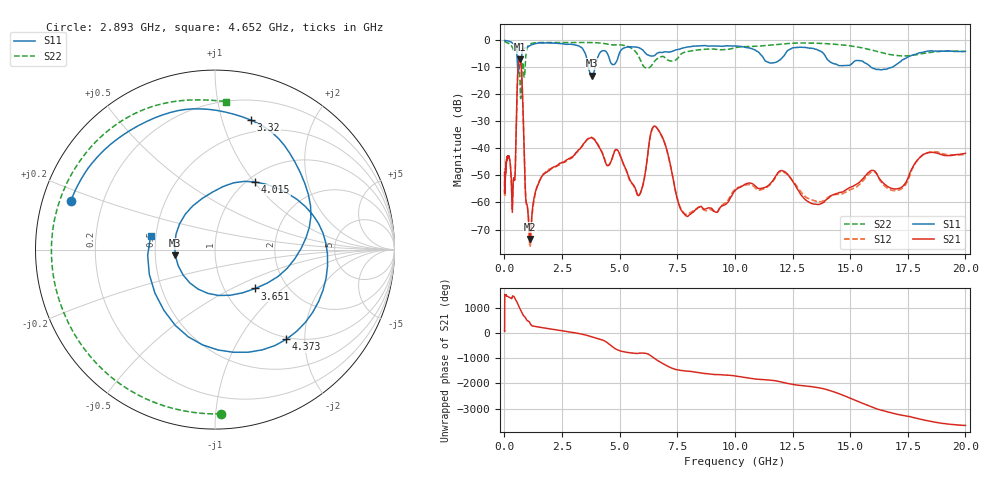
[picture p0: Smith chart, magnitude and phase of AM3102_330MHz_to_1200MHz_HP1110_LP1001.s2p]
! Date/Time: Tue, Sep 11, 2018 5:23 PM
! Network Analyzer: Agilent Technologies E8362B Rev: A.07.50.63
! Sweep from 0.010 to 20.000 GHz, 1601 Points, Sweep Type: LOG
! Power Supply: 4.949 V, 0.001 A
# Hz S DB R 50
!freq MagS11 AngS11 MagS21 AngS21 MagS12 AngS12 MagS22 AngS22
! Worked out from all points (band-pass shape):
!   1601 points, 10 MHz to 20 GHz, reference 50 ohm
!   highest |S21| = -6.95 dB at 672.9 MHz (marker M1); lowest = -73.5 dB at 1.119 GHz (marker M2)
!   |S21| within 3 dB of the highest: 594.6 MHz to 733 MHz (138.4 MHz wide, 20.9 % of centre)
!   lowest |S11| = -13.0 dB at 3.811 GHz (marker M3), VSWR 1.58, Z = 31.8 - j2.16 ohm
!   |S11| at or under -10 dB: 573.3 MHz to 630.7 MHz (57.46 MHz wide, 9.54 % of centre); 3.649 GHz to 3.937 GHz (288.1 MHz wide, 7.59 % of centre); 15.91 GHz to 16.8 GHz (881.1 MHz wide, 5.39 % of centre)
!   |S22| runs from -21.5 to -0.2 dB; largest |S21 - S12| = 0.006
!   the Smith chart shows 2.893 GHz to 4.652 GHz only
!   S11 on the Smith chart (normalised r, x): 2.893 GHz: 0.08, +0.16; 3.32 GHz: 0.38, +1.24; 3.651 GHz: 1.39, -0.67; 4.015 GHz: 1.09, +1.01; 4.373 GHz: 0.97, -1.63; 4.652 GHz: 0.47, +0.08
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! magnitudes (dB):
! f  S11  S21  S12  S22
! 10 MHz  0.0  -48.9  -55.2  -0.2
! 35.55 MHz  -0.1  -51.3  -51.2  -0.5
! 126.4 MHz  -0.2  -43.3  -43.4  -0.9
! 259 MHz  -0.5  -46.1  -46.3  -1.5
! 339.5 MHz  -1.0  -63.3  -62.2  -2.5
! 447.2 MHz  -1.8  -51.8  -51.5  -3.8
! 578 MHz  -10.7  -12.5  -12.5  -4.7
! 672.9 MHz  -9.2  -7.0  -7.0  -14.2
! 925.1 MHz  -2.8  -58.2  -58.2  -6.3
! 1.119 GHz  -1.9  -73.5  -75.9  -1.3
! 1.59 GHz  -1.0  -50.7  -50.9  -0.8
! 2.893 GHz  -1.4  -43.6  -43.3  -0.8
! 3.32 GHz  -2.5  -39.7  -39.7  -0.8
! 3.651 GHz  -10.1  -36.3  -36.1  -0.8
! 3.811 GHz  -13.0  -36.2  -36.0  -0.8
! 4.015 GHz  -7.2  -38.1  -37.9  -0.9
! 4.373 GHz  -3.9  -44.9  -44.7  -1.2
! 4.652 GHz  -8.7  -44.2  -44.2  -1.7
! 5.652 GHz  -2.4  -54.2  -54.6  -3.8
! 6.58 GHz  -5.1  -32.0  -32.1  -7.1
! 7.958 GHz  -2.4  -65.2  -64.3  -4.1
! 20 GHz  -4.1  -41.8  -42.4  -4.0
